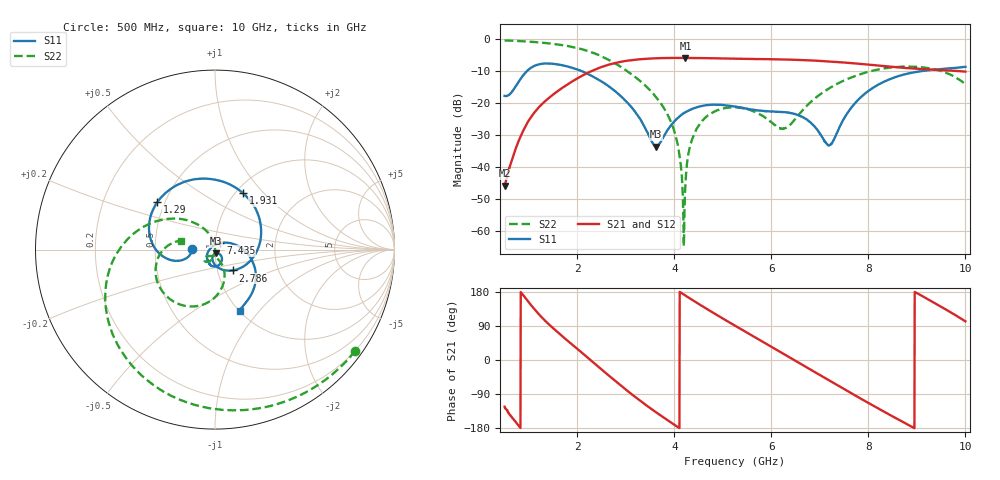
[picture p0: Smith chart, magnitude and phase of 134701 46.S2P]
!  2-Port S-parameters saved by WinCal
! VAR MeasName=S-Parameters (CALIBRATED_DATA) read from VNA (N5242A)
! VAR MeasDate=2013-7-3 16:38:19
! VAR NAME=134701 46
! VAR FILENAME=134701 46.S2P
! VAR DATE=2013-7-3 16:38:19
! VAR PHYS_PORTS=1,2
# Hz S MA R 50
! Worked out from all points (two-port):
!   1601 points, 500 MHz to 10 GHz, reference 50 ohm
!   highest |S21| = -5.79 dB at 4.229 GHz (marker M1); lowest = -45.9 dB at 500 MHz (marker M2)
!   |S21| within 3 dB of the highest: 2.474 GHz to 8.634 GHz (6.159 GHz wide, 111 % of centre)
!   lowest |S11| = -33.6 dB at 3.623 GHz (marker M3), VSWR 1.04, Z = 50.5 - j2.04 ohm
!   |S11| at or under -10 dB: start of sweep to 957.3 MHz; 2.098 GHz to 9.07 GHz (6.972 GHz wide, 125 % of centre)
!   |S22| runs from -64.9 to -0.3 dB; largest |S21 - S12| = 0.0031
!   S11 on the Smith chart (normalised r, x): 500 MHz: 0.77, +0.01; 1.29 GHz: 0.46, +0.29; 1.931 GHz: 1.08, +0.77; 2.786 GHz: 1.18, -0.28; 7.435 GHz: 1.06, +0.08; 10 GHz: 1.00, -0.80
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5e8  0.1299 178.5  0.005086 -123.3  0.005084 -124.7  0.9628 -35.9
8.740625e8  0.2679 -168.7  0.0357 172.6  0.03568 172.4  0.9355 -62.3
1.289688e9  0.4162 140.5  0.09979 109.5  0.0995 109.3  0.885 -91.6
1.930938e9  0.3505 63.6  0.2278 36.6  0.2272 36.6  0.7519 -137.3
2.085312e9  0.3191 44.3  0.2663 20.1  0.2655 20.1  0.7043 -148.6
2.785938e9  0.1525 -49.7  0.4276 -55.9  0.4278 -55.9  0.4179 162.3
3.623125e9  0.0208 -75.7  0.5053 -138.1  0.5055 -138.0  0.1247 116.5
3.670625e9  0.02231 -63.0  0.5074 -142.4  0.5071 -142.3  0.1122 114.3
4.003125e9  0.05205 -46.4  0.512 -171.3  0.5126 -171.3  0.03556 97.2
4.104062e9  0.06181 -51.4  0.5122 -179.7  0.5121 -179.7  0.01551 92.1
4.175312e9  0.06806 -55.4  0.5132 174.3  0.5128 174.4  0.003277 87.3
4.22875e9  0.07204 -58.8  0.5132 170.0  0.5127 169.9  0.005883 -79.7
4.305938e9  0.07733 -63.3  0.512 163.6  0.5119 163.7  0.01852 -91.7
4.478125e9  0.08674 -73.5  0.5099 149.8  0.5105 149.8  0.04183 -101.4
5.25e9  0.0884 -108.5  0.4984 90.6  0.4988 90.6  0.08621 -131.4
6.241562e9  0.07265 -121.5  0.4845 17.0  0.4847 17.1  0.03976 -105.7
6.835312e9  0.04738 -153.4  0.4678 -27.4  0.4675 -27.4  0.1084 -65.3
7.191562e9  0.0218 125.0  0.4512 -54.0  0.4511 -54.1  0.1709 -72.1
7.435e9  0.04696 50.8  0.4383 -72.2  0.4379 -72.2  0.2153 -79.7
8.420625e9  0.2342 -21.8  0.376 -143.3  0.3752 -143.2  0.3591 -120.2
9.245938e9  0.3286 -54.3  0.3384 159.1  0.3391 159.3  0.3536 -159.4
1e10  0.3715 -67.9  0.3129 102.2  0.3137 102.4  0.1985 165.5
